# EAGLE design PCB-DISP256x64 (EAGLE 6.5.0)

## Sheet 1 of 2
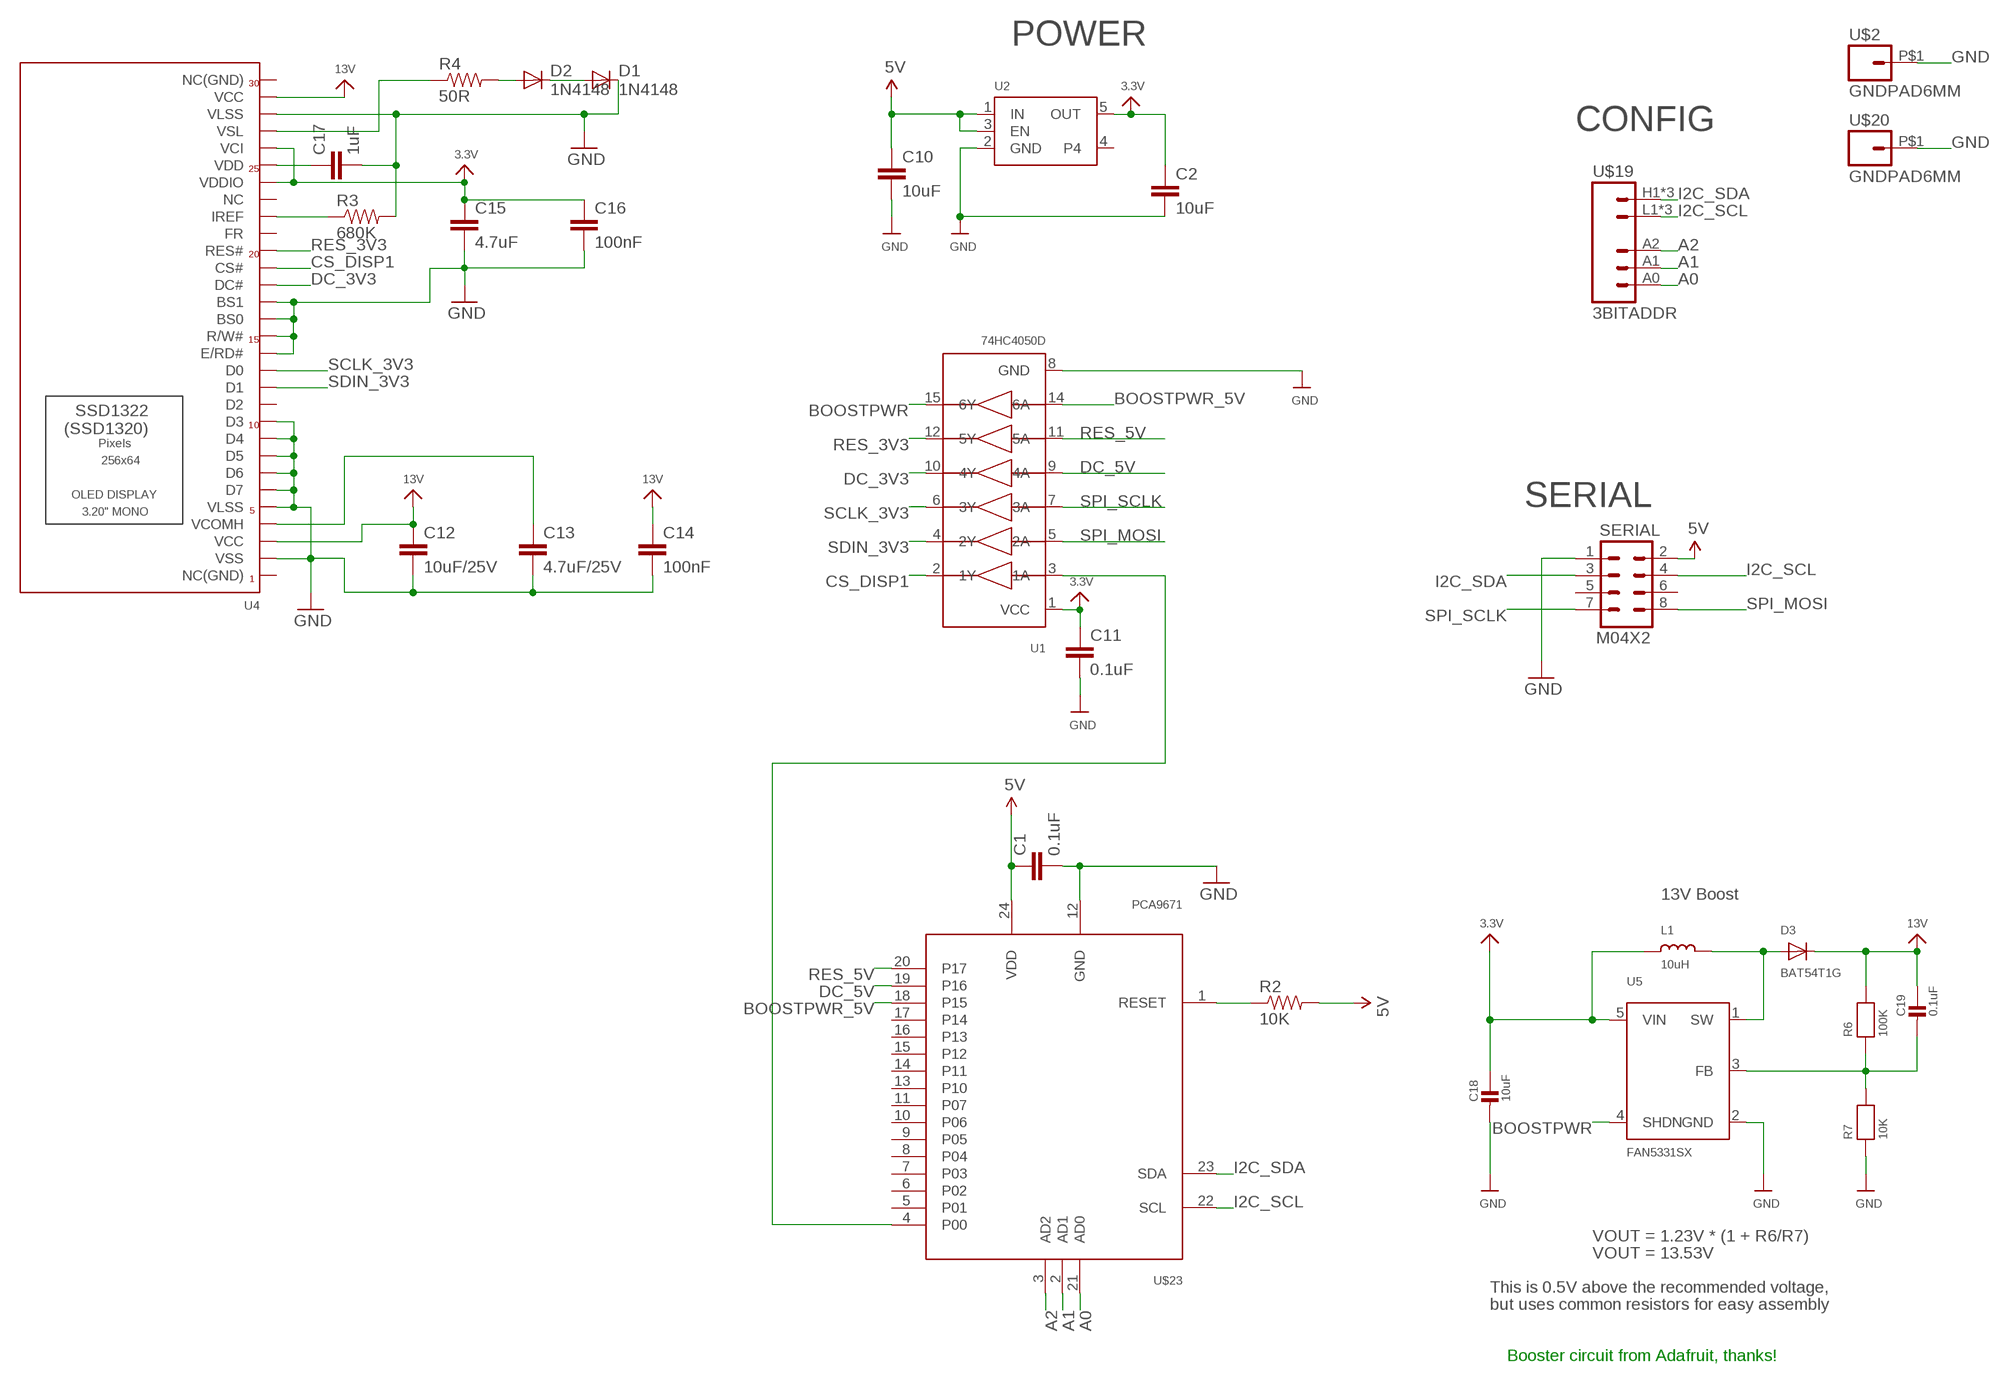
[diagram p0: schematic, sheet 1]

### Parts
C1  0.1uF  CAP0603-CAP  [0603-CAP]
C2  10uF  CAP0805  [0805]
C10  10uF  CAP0805  [0805]
C11  0.1uF  CAP0603-CAP  [0603-CAP]
C12  10uF/25V  CAP0805  [0805]
C13  4.7uF/25V  CAP0805  [0805]
C14  100nF  CAP0603-CAP  [0603-CAP]
C15  4.7uF  CAP0805  [0805]
C16  100nF  CAP0603-CAP  [0603-CAP]
C17  1uF  CAP0603-CAP  [0603-CAP]
C18  10uF  CAP_CERAMIC0805  [0805]
C19  0.1uF  CAP_CERAMIC0603  [0603]
D1  1N4148  DIODESOD  [SOD-323]
D2  1N4148  DIODESOD  [SOD-323]
D3  BAT54T1G  DIODESOD-123  [SOD-123]
L1  10uH  INDUCTOR  [INDUCTOR_1007]
R2  10K  RESISTOR0603-RES  [0603-RES]
R3  680K  RESISTOR0603-RES  [0603-RES]
R4  50R  RESISTOR0603-RES  [0603-RES]
R6  100K  RESISTOR0603  [0603]
R7  10K  RESISTOR0603  [0603]
SERIAL  M04X2  [2X4]
U1  74HC4050D  74HC4050DTSSOP16  [TSSOP16]
U2  VREG_SOT23-5  [SOT23-5]
U4  ER_OLED032-1TOP  [FPC_XF2M-3015-1A]
U5  FAN5331SX  FAN5331  [SOT23-5@1]
U$2  GNDPAD6MM  [3.2MMPAD6MM]
U$19  3BITADDR  [3BITADDR]
U$20  GNDPAD6MM  [3.2MMPAD6MM]
U$23  PCA9671  [TSSOP24]

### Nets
3.3V [Power]: C2.1 C11.1 C15.1 C16.1 C18.1 L1.P$1 U1.1(VCC) U2.5(OUT) U4.P$5(VCI) U4.P$7(VDDIO) U5.5(VIN)
5V [Power]: C1.1 C10.1 R2.2 SERIAL.2 U2.1(IN) U2.3(EN) U$23.24(VDD)
13V [Power]: C12.1 C14.1 C19.1 D3.C R6.2 U4.P$2(VCC) U4.P$28(VCC)
A0: U$19.A0 U$23.21(AD0)
A1: U$19.A1 U$23.2(AD1)
A2: U$19.A2 U$23.3(AD2)
BOOSTPWR: U1.15(6Y) U5.4(SHDN)
BOOSTPWR_5V [Power]: U1.14(6A) U$23.18(P15)
CS_DISP1: U1.2(1Y) U4.P$12(CS#)
DC_3V3: U1.10(4Y) U4.P$13(DC#)
DC_5V: U1.9(4A) U$23.19(P16)
GND [Power]: C1.2 C2.2 C10.2 C11.2 C12.2 C13.2 C14.2 C15.2 C16.2 C17.2 C18.2 D1.1(C) R3.2 R7.1 SERIAL.1 U1.8(GND) U2.2(GND) U4.P$3(VLSS) U4.P$14(BS1) U4.P$15(BS0) U4.P$16(R/W#) U4.P$17(E/RD#) U4.P$21(D3) U4.P$22(D4) U4.P$23(D5) U4.P$24(D6) U4.P$25(D7) U4.P$26(VLSS) U4.P$29(VSS) U5.2(GND) U$2.P$1 U$20.P$1 U$23.12(GND)
I2C_SCL: SERIAL.4 U$19.L1(GND) U$19.L2(GND) U$19.L3(GND) U$23.22(SCL)
I2C_SDA: SERIAL.3 U$19.H1(VCC) U$19.H2(VCC) U$19.H3(VCC) U$23.23(SDA)
N$1: R2.1 U$23.1(RESET)
N$3: U1.3(1A) U$23.4(P00)
N$5: C13.1 U4.P$27(VCOMH)
N$6: R4.1 U4.P$4(VSL)
N$10: R3.1 U4.P$9(IREF)
N$11: D2.2(A) R4.2
N$12: C17.1 U4.P$6(VDD)
N$13: D1.2(A) D2.1(C)
N$14 [BoostPower]: D3.A L1.P$2 U5.1(SW)
N$15: C19.2 R6.1 R7.2 U5.3(FB)
RES_3V3: U1.12(5Y) U4.P$11(RES#)
RES_5V: U1.11(5A) U$23.20(P17)
SCLK_3V3: U1.6(3Y) U4.P$18(D0)
SDIN_3V3: U1.4(2Y) U4.P$19(D1)
SPI_MOSI: SERIAL.8 U1.5(2A)
SPI_SCLK: SERIAL.7 U1.7(3A)
Unconnected: SERIAL.5 SERIAL.6 U2.4 U4.P$1(NC(GND)) U4.P$8(NC) U4.P$10(FR) U4.P$20(D2) U4.P$30(NC(GND)) U$23.5(P01) U$23.6(P02) U$23.7(P03) U$23.8(P04) U$23.9(P05) U$23.10(P06) U$23.11(P07) U$23.13(P10) U$23.14(P11) U$23.15(P12) U$23.16(P13) U$23.17(P14)

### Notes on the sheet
- POWER
- CONFIG
- SERIAL
- 13V Boost
- VOUT = 1.23V * (1 + R6/R7)
- VOUT = 13.53V
- This is 0.5V above the recommended voltage,
- but uses common resistors for easy assembly
- Booster circuit from Adafruit, thanks!

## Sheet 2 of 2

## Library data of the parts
C1 C2 C10-C17 = SparkFun:CAP: Capacitor
C18 C19 = microbuilder:CAP_CERAMIC: Ceramic Capacitors
D1 D2 = SparkFun:DIODE: Diode
D3 = microbuilder:DIODE: Diode
L1 = microbuilder:INDUCTOR: Inductors
R2-R4 = SparkFun:RESISTOR: Resistor
R6 R7 = microbuilder:RESISTOR: Resistors
SERIAL = SparkFun:M04X2
U1 = SKAARHOJ:74HC4050D: 6-channel level shifter 74HC4050D - 2V-6V Supply Digikey: 74HC4050D,653-ND Mouser: 771-74HC4050D-T
U2 = microbuilder:VREG_SOT23-5: SOT23-5 Fixed Voltage Regulators To better organise some of the SOT23-5 fixed voltage regulators in this library, this new part was created. Part Current Out V Out V In V Dropout Digikey Part No. ADP121 150mA 3.3V 3.4-5.5V 0.09V @ 150mA ADP121-AUJZ33R7CT-ND ADP121 150mA 3.0V 3.1-5.5V 0.09V @ 150mA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
U4 = SKAARHOJ:ER_OLED032-1: 128x128 1.5" RGB OLED - UG-2828GDEDF11 30-Pin 0.5mm Pitch FPC Cable (Top+Bottom Contacts) - OMRON XF2M-3015-1A (Digikey: OR723TR-ND) This FPC connector has contacts on the top and bottom, but the appropriate pin needs to be selected depending on whether the OLED will be inserted right-side up (use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
U5 = microbuilder:FAN5331: FAN5331 - LED/OLED 20V Boost Converter Digikey: FAN5331SXCT-ND
U$2 U$20 = SKAARHOJ:GNDPAD
U$19 = SKAARHOJ:3BITADDR
U$23 = SKAARHOJ:PCA9671

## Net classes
0 default: width 0.203 mm, drill 0.406 mm, clearance 0.152 mm
1 Power: width 0.305 mm, drill 0.61 mm, clearance 0.152 mm
2 BoostPower: width 0.61 mm, drill 0.61 mm, clearance 0.305 mm

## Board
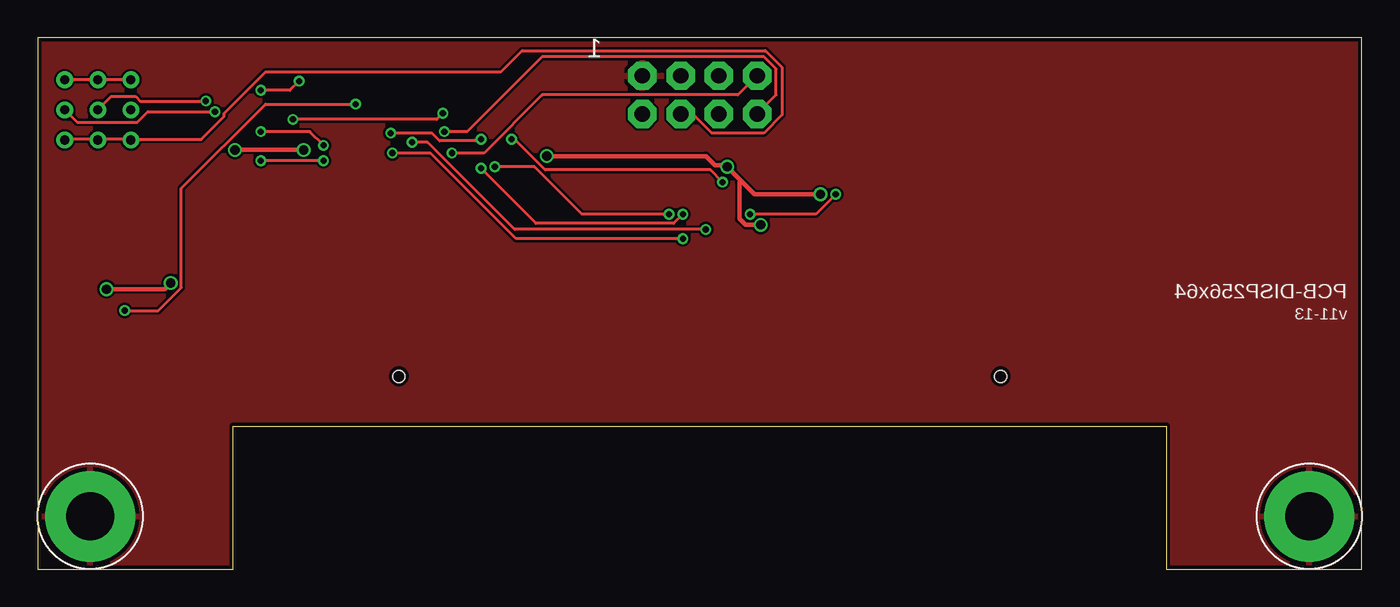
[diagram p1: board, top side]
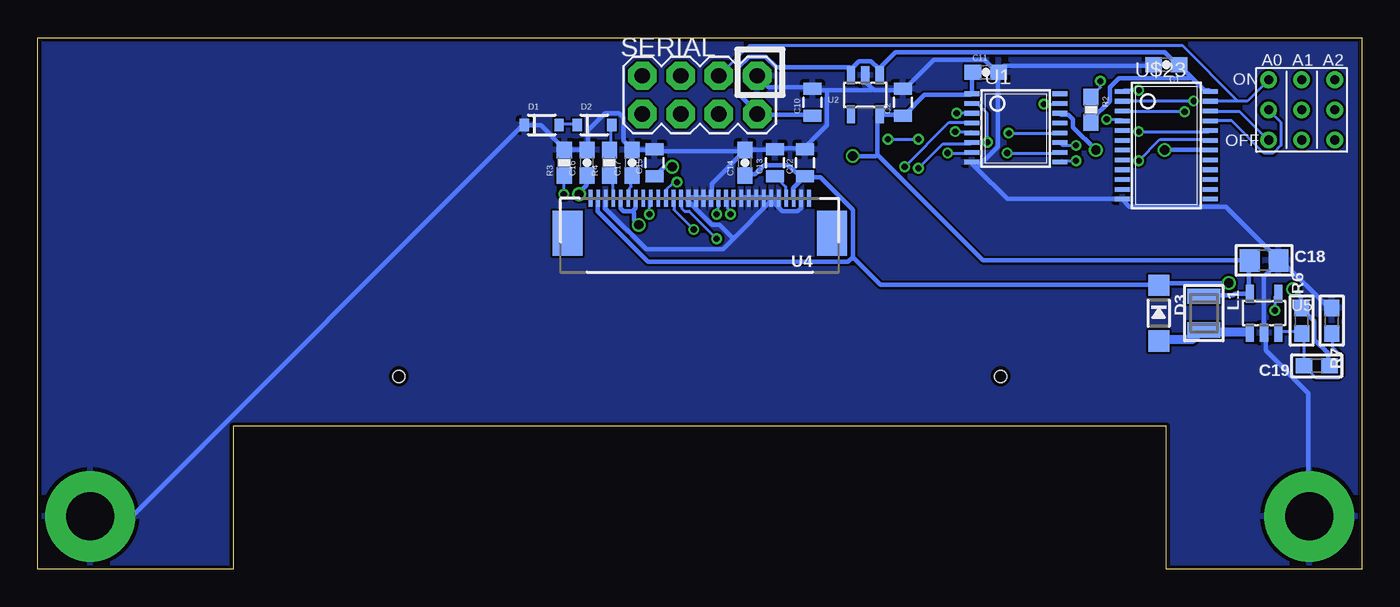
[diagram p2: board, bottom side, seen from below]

Size 88 x 35.3 mm. Coordinates in mm from the lower left corner, seen from the top.
Outline: 88,0 88,35.3 0,35.3 0,0 13,0 13,9.5 75,9.5 75,0 88,0
Copper layers (1*16): Top 0.035mm / dielectric 1.5mm / Bottom 0.035mm
Design rules "Fusion_eagle_rule_v1.1": minimum track width 6mil, minimum drill 12mil, track to track 6mil, track to pad 6mil, pad to pad 6mil, via to via 6mil, smd to smd 0mil, copper to edge 10mil, drill to drill 10mil, minimum pad ring 10mil, minimum via ring 6mil, stop-mask expansion 2mil, vias tented up to drill 100mil, thermal gap 10mil
Holes 0.8 mm at 24,12.8 64,12.8

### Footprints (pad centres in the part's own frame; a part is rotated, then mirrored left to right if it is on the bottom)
0603-CAP = smd 1.1 x 1: 1 -0.85,0; 2 0.85,0
0805 = smd 0.8 x 1.2: 1 -0.9,0; 2 0.9,0
0805' = smd 1.3 x 1.5: 1 -0.95,0; 2 0.95,0
0603 = smd 1.1 x 1: 1 -0.85,0; 2 0.85,0
SOD-323 = smd 0.63 x 0.83: 1 -1.15,0; 2 1.15,0
SOD-123 = smd 1.4 x 1.4: A 1.85,0; C -1.85,0
INDUCTOR_1007 = smd 1.016 x 2.2: P$1 -1.127,0; P$2 1.127,0
0603-RES = smd 1.1 x 1: 1 -0.85,0; 2 0.85,0
2X4 = drill 1.016 pad 1.88 octagon: 1 -3.81,-1.27; 2 -3.81,1.27; 3 -1.27,-1.27; 4 -1.27,1.27; 5 1.27,-1.27; 6 1.27,1.27; 7 3.81,-1.27; 8 3.81,1.27
TSSOP16 = smd 0.305 x 0.991: 1 -3.575,-2.918; 2 -2.925,-2.918; 3 -2.275,-2.918; 4 -1.625,-2.918; 5 -0.975,-2.918; 6 -0.325,-2.918; 7 0.325,-2.918; 8 0.975,-2.918; 9 0.975,2.918; 10 0.325,2.918; 11 -0.325,2.918; 12 -0.975,2.918; 13 -1.625,2.918; 14 -2.275,2.918; 15 -2.925,2.918; 16 -3.575,2.918
SOT23-5 = smd 0.55 x 1.2: 1 -0.95,-1.3; 2 0,-1.3; 3 0.95,-1.3; 4 0.95,1.3; 5 -0.95,1.3
FPC_XF2M-3015-1A = smd 0.25 x 1.1: P$1 7.25,-2.63; P$2 6.75,-2.63; P$3 6.25,-2.63; P$4 5.75,-2.63; P$5 5.25,-2.63; P$6 4.75,-2.63; P$7 4.25,-2.63; P$8 3.75,-2.63; P$9 3.25,-2.63; P$10 2.75,-2.63; P$11 2.25,-2.63; P$12 1.75,-2.63; P$13 1.25,-2.63; P$14 0.75,-2.63; P$15 0.25,-2.63; P$16 -0.25,-2.63; P$17 -0.75,-2.63; P$18 -1.25,-2.63; P$19 -1.75,-2.63; P$20 -2.25,-2.63; P$21 -2.75,-2.63; P$22 -3.25,-2.63; P$23 -3.75,-2.63; P$24 -4.25,-2.63; P$25 -4.75,-2.63; P$26 -5.25,-2.63; P$27 -5.75,-2.63; P$28 -6.25,-2.63; P$29 -6.75,-2.63; P$30 -7.25,-2.63 | smd 2 x 3: SUPPORT1 8.79,-0.305; SUPPORT2 -8.79,-0.305
SOT23-5@1 = smd 0.55 x 1.2: 1 -0.95,-1.3; 2 0,-1.3; 3 0.95,-1.3; 4 0.95,1.3; 5 -0.95,1.3
3.2MMPAD6MM = drill 3.2 pad 6: P$1 0,0
3BITADDR = drill 0.6: A0 -2.2,0; A1 0,0; A2 2.2,0; H1 -2.2,2; H2 0,2; H3 2.2,2; L1 -2.2,-2; L2 0,-2; L3 2.2,-2
TSSOP24 = smd 0.305 x 0.991: 1 -4.225,-2.918; 2 -3.575,-2.918; 3 -2.925,-2.918; 4 -2.275,-2.918; 5 -1.625,-2.918; 6 -0.975,-2.918; 7 -0.325,-2.918; 8 0.325,-2.918; 9 0.975,-2.918; 10 1.625,-2.918; 11 2.275,-2.918; 12 2.925,-2.918; 13 2.925,2.918; 14 2.275,2.918; 15 1.625,2.918; 16 0.975,2.918; 17 0.325,2.918; 18 -0.325,2.918; 19 -0.975,2.918; 20 -1.625,2.918; 21 -2.275,2.918; 22 -2.925,2.918; 23 -3.575,2.918; 24 -4.225,2.918

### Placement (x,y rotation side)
C1  13,33.5 180 bottom
C2  30.5,31 90 bottom
C10  36.5,31 90 bottom
C11  25,33 0 bottom
C12  37,27 90 bottom
C13  39,27 90 bottom
C14  41,27 90 bottom
C15  47,27 90 bottom
C16  51.5,27 90 bottom
C17  48.5,27 90 bottom
C18  10uF  [0805']  6.5,20.5 0 bottom
C19  3,13.5 180 bottom
D1  54.5,29.5 0 bottom
D2  51,29.5 0 bottom
D3  13.5,17 270 bottom
L1  10.5,17 270 bottom
R2  18,30.5 270 bottom
R3  53,27 90 bottom
R4  50,27 90 bottom
R6  4,16.5 90 bottom
R7  2,16.5 270 bottom
SERIAL  44,31.5 180 bottom
U1  23,28 270 bottom
U2  33,31.5 180 bottom
U4  44,22 180 bottom
U5  6.5,17 0 bottom
U$2  3.5,3.5 0 top
U$19  4,30.5 0 bottom
U$20  84.5,3.5 0 top
U$23  13,27.5 270 bottom

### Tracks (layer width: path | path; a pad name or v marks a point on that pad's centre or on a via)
3.3V  (via drill 0.61)
  Top 0.305: v52.02,24.89 47.65,24.89 46.74,25.81 | 46.74,25.81 v45.82,26.72 45.72,26.82 45.01,26.82 44.4,27.43 v33.83,27.43 | v48.06,22.86 47.04,22.86 46.63,23.27 46.63,25.7 46.74,25.81
  Bottom 0.305: 48.46,23.77 48.26,23.98 48.26,24.59 U4.P$7 | 48.46,23.77 49.07,23.77 49.28,23.98 49.28,24.59 U4.P$5 | v52.02,24.89 52.02,24.99 51.51,25.5 51.51,26.11 C16.1 | v45.82,26.72 46.33,26.72 46.94,26.11 C15.1 | v48.06,22.86 48.36,23.16 48.36,23.67 48.46,23.77 | L1.P$1 10.46,18.19 8.53,18.19 8.43,18.29 7.62,18.29 U5.5 7.52,18.39 7.52,20.42 C18.1 7.62,20.52 25.2,20.52 32.21,27.53 | C11.1 25.91,32.92 25.91,31.6 U1.1 26.01,31.5 29.06,31.5 30.38,30.18 C2.1 30.58,30.18 32,30.18 U2.5 32.11,30.07 32.21,29.97 32.21,27.53 | v33.83,27.43 32.31,27.43 32.21,27.53
5V
  Bottom 0.305: 11.38,32.72 12.09,33.43 C1.1 12.29,33.53 13.11,34.34 30.99,34.34 32,33.33 U2.1 32.11,32.82 32.11,33.22 32.61,33.73 33.43,33.73 33.93,33.22 33.93,32.82 U2.3 34.04,33.33 38.91,33.33 39.62,34.04 40.74,34.04 41.45,33.33 41.45,31.6 40.23,30.38 SERIAL.2 40.13,30.18 36.58,30.18 C10.1 | 11.38,32.72 10.46,31.8 10.16,31.8 U$23.24 | R2.2 17.98,29.67 17.98,29.87 16.76,31.09 16.76,32 16.15,32.61 11.48,32.61 11.38,32.72
13V  (via drill 0.61)
  Top 0.305: v4.57,18.59 8.43,18.59 v8.84,19
  Bottom 0.305: C19.1 2.23,13.51 2.23,14.33 3.15,15.24 3.15,16.46 3.96,17.27 R6.2 4.06,17.48 4.06,18.09 v4.57,18.59 | U4.P$28 37.8,24.69 37.8,25.3 37.08,26.01 C12.1 | C14.1 40.95,26.21 40.34,26.21 39.73,26.82 38.1,26.82 37.29,26.01 C12.1 | 33.83,20.73 34.14,20.42 47.45,20.42 50.8,23.77 50.8,24.59 U4.P$2 | 33.83,20.73 33.83,23.88 35.97,26.01 36.88,26.01 C12.1 | 33.83,20.73 32,18.9 13.51,18.9 D3.C 13.41,19 v8.84,19
A0
  Bottom 0.203: U$23.21 10.06,29.77 8.64,29.77 6.5,27.64 5.89,27.64 5.38,28.14 5.38,29.67 6.2,30.48 U$19.A0
A1  (via drill 0.41)
  Top 0.203: v11.18,31.09 6.81,31.09 6.5,31.39 4.88,31.39 4.06,30.58 U$19.A1
  Bottom 0.203: v11.18,31.09 15.85,31.09 U$23.2
A2  (via drill 0.41)
  Top 0.203: v11.79,30.38 7.32,30.38 6.6,29.67 2.64,29.67 1.83,30.48 U$19.A2
  Bottom 0.203: v11.79,30.38 15.85,30.38 U$23.3
BOOSTPWR  (via drill 0.41)
  Top 0.203: v21.13,30.89 15.14,30.89 9.55,25.3 9.55,18.69 8.03,17.17 v5.79,17.17
  Bottom 0.203: v21.13,30.89 20.12,30.89 U1.15 | v5.79,17.17 5.79,18.09 5.59,18.29 U5.4
BOOSTPWR_5V  (via drill 0.61)
  Top 0.305: v17.68,27.84 v13.11,27.84
  Bottom 0.305: v13.11,27.84 10.16,27.84 U$23.18 | v17.68,27.84 19.2,29.36 19.2,29.87 19.51,30.18 20.02,30.18 U1.14
CS_DISP1  (via drill 0.41)
  Top 0.203: v24.89,28.35 25.91,28.35 31.7,22.55 v44.4,22.55
  Bottom 0.203: v24.89,28.35 24.89,30.28 25.5,30.89 25.91,30.89 U1.2 | v44.4,22.55 45.72,23.88 45.72,24.59 U4.P$12
DC_3V3  (via drill 0.41)
  Top 0.203: v23.57,27.64 26.11,27.64 31.8,21.95 v42.88,21.95
  Bottom 0.203: v23.57,27.64 20.12,27.64 U1.10 | v42.88,21.95 44.7,23.77 45.01,23.77 45.21,23.98 45.21,24.59 U4.P$13
DC_5V  (via drill 0.41)
  Top 0.203: v19,27.13 v14.83,27.13
  Bottom 0.203: v14.83,27.13 13.41,28.55 10.16,28.55 U$23.19 | v19,27.13 19.91,27.13 20.02,27.03 U1.9
GND
  Bottom 0.305: R7.1 2.03,17.37 2.23,17.37 5.28,20.42 5.49,20.42 C18.2 | C18.2 5.59,20.32 6.5,19.41 6.5,15.75 U5.2 6.4,15.65 6.4,14.53 3.56,11.68 3.56,3.56 U$2.P$1 | 25.6,26.62 25.91,26.92 U1.8 | 25.6,26.62 23.57,24.59 15.95,24.59 U$23.12 15.85,24.49 15.44,24.08 9.04,24.08 5.59,20.62 C18.2 | 25.6,26.62 24.18,28.04 24.18,32.92 C11.2 | C1.2 13.92,33.43 23.77,33.43 24.08,33.12 C11.2 | 32.51,31.9 32.92,32.31 32.92,32.72 U2.2 | 32.51,31.9 32.41,31.8 30.58,31.8 C2.2 30.38,31.9 28.45,33.83 25.09,33.83 24.28,33.02 C11.2 | 35.56,31.8 32.61,31.8 32.51,31.9 | 35.56,31.8 36.47,31.8 C10.2 36.58,32 39.42,32 40.13,32.72 SERIAL.1 | 39.32,24.59 39.06,24.33 | 39.06,24.33 38.51,23.77 37.49,23.77 37.29,23.98 37.29,24.59 U4.P$29 | 39.32,24.59 U4.P$25 39.32,24.38 41.76,21.95 | 39.06,24.33 38.81,24.59 U4.P$26 | 39.32,24.59 39.42,24.69 39.73,24.69 U4.P$24 39.83,24.69 40.23,24.69 U4.P$23 40.34,24.69 40.74,24.69 U4.P$22 40.84,24.69 41.25,24.69 U4.P$21 | 41.76,21.95 42.47,21.23 47.55,21.23 50.29,23.98 50.29,24.59 U4.P$3 | C14.2 40.95,27.84 39.01,27.84 C13.2 38.91,27.94 37.08,27.94 C12.2 36.98,28.04 35.56,29.46 35.56,31.8 | C14.2 41.05,27.74 43.18,25.6 43.18,24.79 U4.P$17 43.28,24.69 43.69,24.69 U4.P$16 43.89,24.69 44.2,24.69 U4.P$15 44.4,24.69 44.7,24.69 U4.P$14 44.81,24.49 43.18,22.86 42.67,22.86 41.76,21.95 | C14.2 41.25,27.74 46.94,27.74 C15.2 47.04,27.84 48.46,27.84 C17.2 48.56,27.94 49.07,28.45 49.07,29.97 49.38,30.28 50.29,30.28 51.41,29.16 51.41,27.94 C16.2 51.51,27.84 52.93,27.84 R3.2 53.03,27.94 54.56,29.46 55.58,29.46 D1.1 55.78,29.46 81.69,3.56 84.43,3.56 U$20.P$1
  pour Bottom: 0,0 88,0 88,35.5 0,35.5
  pour Top: 0,0 88,0 88,35.5 0,35.5
I2C_SCL
  Top 0.203: U$19.L3 1.83,28.55 3.96,28.55 U$19.L2 4.06,28.55 6.2,28.55 U$19.L1 6.3,28.55 10.87,28.55 12.39,30.07 12.39,30.28 15.14,33.02 30.79,33.02 32.21,34.44 48.36,34.44 49.48,33.33 49.48,30.18 48.26,28.96 44.81,28.96 43.59,30.18 42.77,30.18 SERIAL.4
  Bottom 0.203: U$23.22 10.06,30.38 8.13,30.38 6.3,28.55 U$19.L1
I2C_SDA
  Top 0.203: U$19.H3 1.83,32.51 3.96,32.51 U$19.H2 4.06,32.51 6.2,32.51 U$19.H1
  Bottom 0.203: 8.23,31.09 7.62,31.09 6.3,32.41 U$19.H1 | 8.23,31.09 10.06,31.09 U$23.23 | 8.23,31.09 11.89,34.75 40.74,34.75 42.67,32.82 SERIAL.3
N$1  (via drill 0.41)
  Top 0.203: v14.83,31.8 16.76,31.8 v17.37,32.41
  Bottom 0.203: v14.83,31.8 15.85,31.8 U$23.1 | v17.37,32.41 17.37,32 17.98,31.39 R2.1
N$3  (via drill 0.41)
  Top 0.203: v16.97,29.87 26.52,29.87 v26.92,30.28
  Bottom 0.203: v16.97,29.87 15.95,29.87 U$23.4 | v26.92,30.28 26.01,30.28 U1.3
N$5
  Bottom 0.203: U4.P$27 38.3,24.69 38.3,25.4 38.91,26.01 C13.1
N$6
  Bottom 0.203: U4.P$4 49.78,24.69 49.78,25.91 49.99,26.11 R4.1
N$10  (via drill 0.41)
  Top 0.203: v47.35,23.57 51.71,23.57 v53.03,24.89
  Bottom 0.203: v47.35,23.57 47.35,24.59 U4.P$9 | v53.03,24.89 53.03,26.11 R3.1
N$11
  Bottom 0.203: D2.2 49.89,29.46 49.89,28.04 49.99,27.94 R4.2
N$12
  Bottom 0.203: C17.1 48.56,26.11 48.56,25.4 48.67,25.3 48.67,24.69 U4.P$6
N$13
  Bottom 0.203: D2.1 52.22,29.57 53.34,29.57 D1.2
N$14
  Bottom 0.61: U5.1 7.52,15.75 10.36,15.75 10.46,15.85 L1.P$2 10.77,15.75 11.28,15.24 13.41,15.24 D3.A
N$15
  Bottom 0.203: R7.2 1.93,15.65 1.93,14.73 1.32,14.12 1.32,12.9 1.52,12.7 3.05,12.7 3.76,13.41 C19.2 3.86,13.51 3.86,15.54 3.96,15.65 R6.1 4.06,15.75 5.49,15.75 U5.3
RES_3V3  (via drill 0.41)
  Top 0.203: v23.47,28.96 26.21,28.96 26.72,28.45 29.36,28.45 v29.46,28.55 | v31.5,28.55 31.7,28.55 33.73,26.52 44.7,26.52 v45.52,25.7
  Bottom 0.203: v23.47,28.96 20.12,28.96 U1.12 | v31.5,28.55 v29.46,28.55 | v45.52,25.7 45.72,25.7 46.23,25.2 46.23,24.69 U4.P$11
RES_5V  (via drill 0.41)
  Top 0.203: v14.83,29.06 18.09,29.06 v19,28.14
  Bottom 0.203: v14.83,29.06 10.16,29.06 U$23.20 | v19,28.14 19.91,28.14 20.02,28.25 U1.11
SCLK_3V3  (via drill 0.41)
  Top 0.203: v29.46,26.62 33.12,22.96 42.27,22.96 v42.88,23.57
  Bottom 0.203: v29.46,26.62 27.84,28.25 26.01,28.25 U1.6 | v42.88,23.57 42.88,23.88 42.77,23.98 42.77,24.59 U4.P$18
SDIN_3V3  (via drill 0.41)
  Top 0.203: v30.38,26.72 33.02,26.72 36.17,23.57 v41.96,23.57
  Bottom 0.203: v30.38,26.72 27.43,29.67 26.01,29.67 U1.4 | v41.96,23.57 41.96,23.77 42.16,23.98 42.16,24.59 U4.P$19
SPI_MOSI  (via drill 0.41)
  Top 0.203: v27.03,29.06 28.55,29.06 33.53,34.04 48.26,34.04 49.07,33.22 49.07,31.5 47.85,30.28 SERIAL.8
  Bottom 0.203: v27.03,29.06 26.01,29.06 U1.5
SPI_SCLK  (via drill 0.41)
  Top 0.203: v27.53,27.64 29.67,27.64 33.53,31.5 46.53,31.5 47.75,32.72 SERIAL.7
  Bottom 0.203: v27.53,27.64 26.01,27.64 U1.7

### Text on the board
_tsilk: 1 | PCB-DISP256x64 | v11-13

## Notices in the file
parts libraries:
SparkFun: Licensing: CC v3.0 Share-Alike You are welcome to use this library for commercial purposes.
